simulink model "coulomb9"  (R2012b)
settings: Solver=ode1  StartTime=0.0  StopTime=100  FixedStep=0.001  MaxStep=0.001  RelTol=1e-3
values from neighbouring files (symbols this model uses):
  c = 2200    [coulomb_1.m]    (also in coulomb_10.m = 0.1; coulomb_11.m = 0; coulomb_2.m; coulomb_3.m)
  FG = 500    [coulomb_1.m]    (also in coulomb_10.m = 10; coulomb_11.m = 10; coulomb_2.m; coulomb_3.m)
  FH = 12    [coulomb_10.m]    (also in coulomb_11.m; coulomb_3.m = 600; coulomb_4.m = 600; position_reg_1.m = 3.956)
  k = 10    [coulomb_10.m]    (also in coulomb_11.m; diff_filter_1.m = 250; diff_filter_2.m = 250; dry_friction_1.m = 2200)
  m = 400    [coulomb_1.m]    (also in coulomb_10.m = 10; coulomb_11.m = 10; coulomb_2.m; coulomb_3.m)
  vstr = 0.1    [coulomb_10.m]    (also in coulomb_11.m; coulomb_3.m = 0.05; coulomb_4.m = 0.01; slip_stick_1.m = 0.01)
undefined symbols (not defined in the file or in its folder): sgn

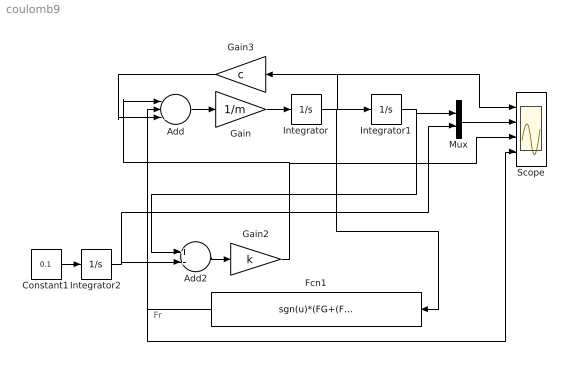
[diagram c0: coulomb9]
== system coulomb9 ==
  note: Fr
  Add : Sum  Inputs=---
  Add2 : Sum  Inputs=+-
  Constant1 : Constant  Value=0.1
  Fcn1 : Fcn  Expr=sgn(u)*(FG+(FH-FG)*exp(-abs(u/vstr)))
  Gain : Gain  Gain=1/m
  Gain2 : Gain  Gain=k
  Gain3 : Gain  Gain=c
  Integrator : Integrator
  Integrator1 : Integrator
  Integrator2 : Integrator
  Mux : Mux  Inputs=2
  Scope : Scope  NumInputPorts=4
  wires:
  Add/1 -> Gain/1
  Gain/1 -> Integrator/1
  Gain3/1 -> Add/3
  Gain2/1 -> Scope/3, Add/1
  Constant1/1 -> Integrator2/1
  Integrator2/1 -> Mux/2, Add2/2
  Add2/1 -> Gain2/1
  Integrator1/1 -> Mux/1, Add2/1
  Integrator/1 -> Integrator1/1, Scope/1, Gain3/1, Fcn1/1
  Mux/1 -> Scope/2
  Fcn1/1 -> Scope/4, Add/2
